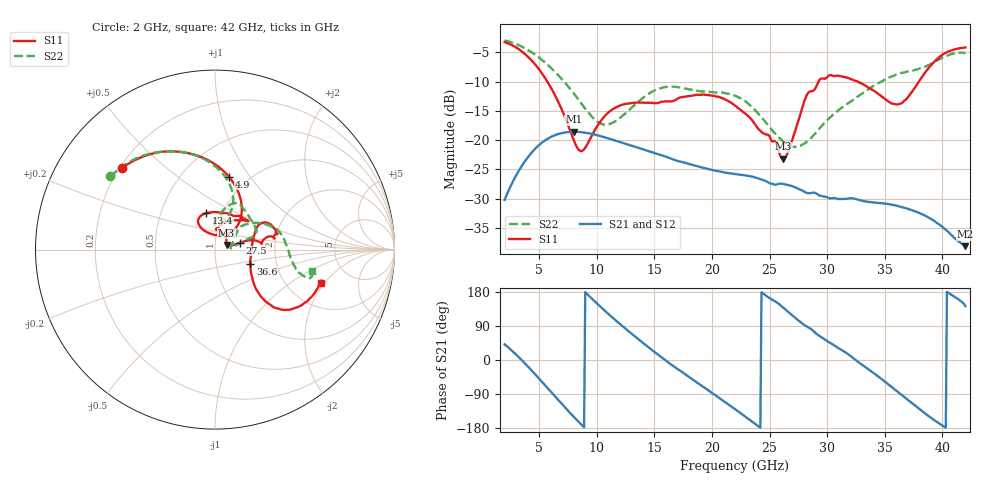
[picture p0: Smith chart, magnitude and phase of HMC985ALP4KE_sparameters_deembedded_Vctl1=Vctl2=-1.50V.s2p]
!s2p File: Measurements: S11, S21, S12, S22
# GHz S dB R 50.0
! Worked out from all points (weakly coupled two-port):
!   401 points, 2 GHz to 42 GHz, reference 50 ohm
!   highest |S21| = -18.58 dB at 8 GHz (marker M1); lowest = -38.1 dB at 42 GHz (marker M2)
!   lowest |S11| = -23.2 dB at 26.2 GHz (marker M3), VSWR 1.15, Z = 56.8 + j2.92 ohm
!   |S11| at or under -10 dB: 5.712 GHz to 29.25 GHz (23.53 GHz wide, 135 % of centre); 32.63 GHz to 37.96 GHz (5.327 GHz wide, 15.1 % of centre)
!   |S22| runs from -21.2 to -3.0 dB; largest |S21 - S12| = 0.00017
!   S11 on the Smith chart (normalised r, x): 2 GHz: 0.21, +0.36; 4.9 GHz: 0.81, +0.80; 13.4 GHz: 0.84, +0.36; 27.5 GHz: 1.32, +0.10; 36.6 GHz: 1.47, -0.24; 42 GHz: 3.08, -1.83
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2  -3.24 138.5  -30.25 41.3  -30.24 41.3  -2.96 145.0
3.4  -4.70 110.5  -24.71 2.4  -24.72 2.4  -3.93 121.9
4.9  -7.66 79.3  -21.01 -46.1  -21.02 -46.1  -5.74 98.2
6.2  -11.67 55.1  -19.30 -90.4  -19.31 -90.4  -7.98 80.6
8  -20.00 56.1  -18.58 -149.9  -18.59 -149.9  -12.01 67.7
8.7  -21.88 86.2  -18.66 -171.8  -18.66 -171.8  -13.85 68.5
10.8  -15.67 122.8  -19.59 127.2  -19.59 127.2  -17.35 87.4
13.4  -13.60 103.4  -21.19 60.1  -21.19 60.0  -13.78 81.8
15.4  -13.60 77.0  -22.46 12.3  -22.47 12.3  -11.21 68.9
18.9  -12.27 41.5  -24.57 -63.6  -24.57 -63.6  -11.61 42.7
22  -14.08 55.7  -25.80 -129.5  -25.80 -129.5  -12.41 20.2
24.5  -18.88 87.3  -26.87 174.3  -26.88 174.3  -16.55 15.1
26.2  -23.18 21.7  -27.51 137.6  -27.52 137.6  -20.29 6.2
27.5  -16.75 15.3  -28.32 104.4  -28.30 104.6  -21.07 7.8
28.2  -12.43 11.7  -29.02 89.1  -29.02 89.1  -20.36 15.6
28.7  -11.61 7.2  -29.01 79.2  -29.01 79.2  -19.42 21.9
31.1  -9.07 19.1  -30.08 29.3  -30.09 29.2  -14.70 41.5
33.3  -10.66 29.9  -30.49 -18.3  -30.49 -18.4  -11.71 34.5
35.4  -13.50 9.4  -30.98 -66.4  -30.99 -66.5  -9.32 22.2
36.6  -13.45 -22.0  -31.51 -95.3  -31.53 -95.3  -8.48 13.7
39.6  -6.06 -42.2  -34.27 -164.8  -34.27 -165.3  -6.35 -14.9
42  -4.16 -17.2  -38.15 142.6  -38.12 142.9  -5.10 -12.4
